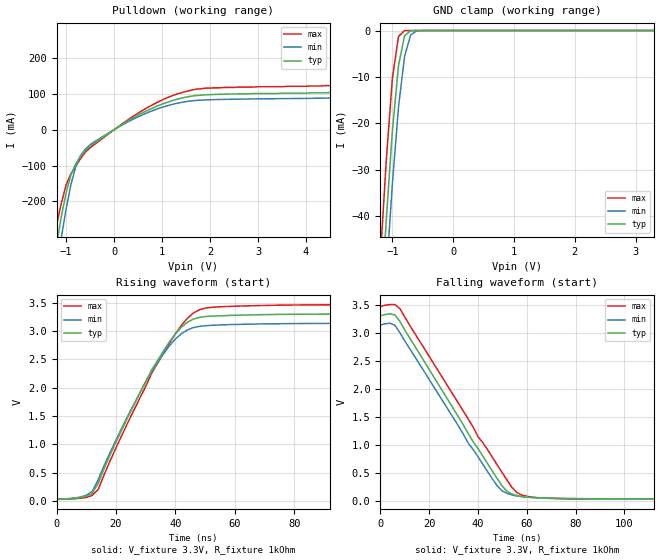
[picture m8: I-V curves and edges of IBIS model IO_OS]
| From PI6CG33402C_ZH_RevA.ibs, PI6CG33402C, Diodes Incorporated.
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[Model]  IO_OS
Model_type  I/O_open_sink
Vinl = 825mV
Vinh = 2.75V
Vmeas =  1.6
Vref = 3.3
Rref = 1k
|Variable   typ   min   max
C_comp   2.23p   2.17p  2.28p
|Variable   typ   min   max
[Voltage Range]   3.3   3.135   3.465
[Temperature Range]   25   85   -40
[GND Clamp Reference]   0   0   0
[Pulldown Reference]   0   0   0
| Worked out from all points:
|   slope of the pulldown table from 0 to 0.495 V, typ, clamps not added: 12.3 ohm
|   GND clamp passes 1 mA (typ) near -0.79 V on its own axis
|   falling waveform, V_fixture 3.3V, R_fixture 1kOhm: 20-80 % time 27.9ns typ, 27ns min, 29.7ns max; typ from 3.3 V to 0.037 V
|   rising waveform, V_fixture 3.3V, R_fixture 1kOhm: 20-80 % time 19ns typ, 18.7ns min, 19.9ns max; typ from 0.037 V to 3.3 V
[GND Clamp]
| Voltage   I(typ)   I(min)   I(max)
-3.3V     -611mA     -617mA     -607mA
-1.2V     -62.2mA    -74.3mA    -49.3mA
-1.1V     -40.5mA    -52.6mA    -27.7mA
-1V       -21.5mA    -32.9mA    -10.2mA
-900mV    -7.54mA    -16.5mA    -1.27mA
-800mV    -1.13mA    -5.57mA    -24.2uA
-700mV    -53.2uA    -958uA     -202nA
-600mV    -1.35uA    -74.3uA    -1.52nA
3.3V      9.9pA      10.4pA     9.9pA
[Pulldown]   |Note: Vtable = Vcc - Voutput
| Voltage   I(typ)   I(min)  I(max)
-3.3V     -2.49A     -2.53A     -2.48A
-1.3V     -409mA     -477mA     -343mA
-1.2V     -322mA     -388mA     -266mA
-1.1V     -242mA     -301mA     -205mA
-800mV    -94.8mA    -103mA     -102mA
-600mV    -57.8mA    -54.1mA    -62.8mA
1.3V      84.6mA     73.4mA     99.1mA
5.7V      114mA      102mA      134mA
5.9V      148mA      169mA      142mA
6.1V      249mA      303mA      225mA
6.2V      323mA      388mA      278mA
6.6V      684mA      754mA      614mA
[Falling Waveform]
V_fixture = 3.3V
V_fixture_min = 3.135V
V_fixture_max = 3.465V
R_fixture = 1kOhm
C_fixture = 0F
|   Time   V(typ)   V(min)   V(max)
0s        3.3V       3.135V     3.465V
4ns       3.336V     3.169V     3.501V
6ns       3.315V     3.132V     3.499V
8ns       3.203V     3.003V     3.43V
36ns      1.208V     1.034V     1.465V
48ns      393.9mV    268.3mV    640.3mV
52ns      174.1mV    138.2mV    371.8mV
58ns      85.35mV    81.93mV    110.2mV
80ns      45.11mV    47.9mV     42.59mV
198ns     36.94mV    39.02mV    34.44mV
[Rising Waveform]
V_fixture = 3.3V
V_fixture_min = 3.135V
V_fixture_max = 3.465V
R_fixture = 1kOhm
C_fixture = 0F
|   Time   V(typ)   V(min)   V(max)
0s        36.71mV    38.75mV    34.24mV
10ns      87.45mV    105.8mV    67.14mV
12ns      138.9mV    172.9mV    102.9mV
14ns      314.9mV    378.3mV    207.2mV
22ns      1.266V     1.294V     1.165V
32ns      2.314V     2.285V     2.255V
40ns      2.949V     2.858V     2.948V
48ns      3.237V     3.079V     3.371V
80ns      3.293V     3.129V     3.456V
198ns     3.3V       3.135V     3.465V
[Ramp]
|   typ   min   max
dV/dt_r   1.57/13.8E-12   1.45/12.9E-12   1.70/15.3E-12
dV/dt_f   1.57/52.9E-12   1.45/54.0E-12   1.70/53.1E-12
R_load =   50.0000
